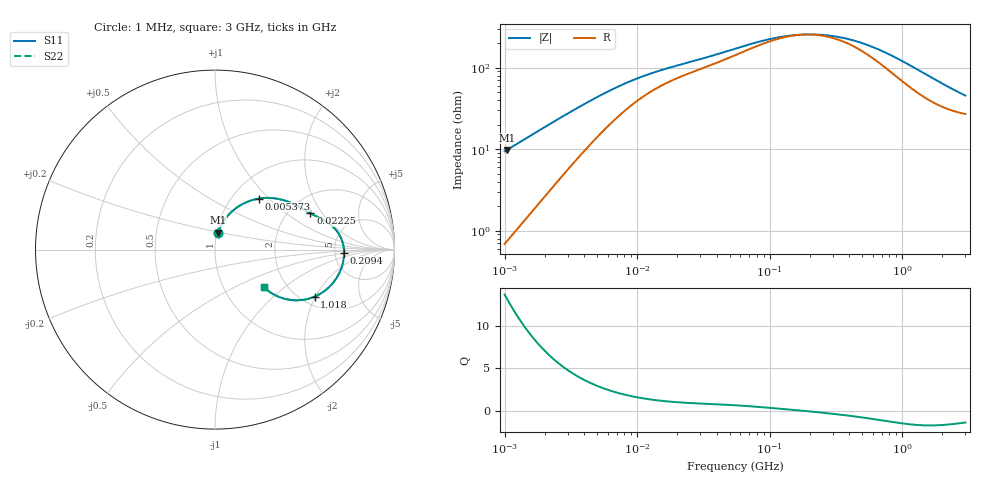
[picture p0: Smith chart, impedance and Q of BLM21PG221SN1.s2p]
! BLM21PG221SN1
# Hz S RI R 50
!Freq.(Hz) S11(Real) S11(Imag) S21(Real) S21(Imag) S12(Real) S12(Imag) S22(Real) S22(Imag)
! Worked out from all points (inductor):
!   401 points, 1 MHz to 3 GHz, reference 50 ohm
!   read as one part in series: L = 1.48 uH near 1.041 MHz
!   highest Q = 13.1 at 1.041 MHz (marker M1), where L = 1.49 uH
!   self-resonance near 183.2 MHz
!   S11 on the Smith chart (normalised r, x): 1 MHz: 1.01, +0.19; 5.373 MHz: 1.32, +0.87; 22.25 MHz: 2.60, +1.56; 209.4 MHz: 6.09, -0.44; 1.018 GHz: 2.34, -1.96; 3 GHz: 1.54, -0.73
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1000000  0.0153 0.0916  0.9847 -0.0916  0.9847 -0.0916  0.0153 0.0916
1040844  0.0166 0.0951  0.9834 -0.0951  0.9834 -0.0951  0.0166 0.0951
2139570  0.0629 0.1787  0.9371 -0.1787  0.9371 -0.1787  0.0629 0.1787
2888807  0.1043 0.221  0.8957 -0.221  0.8957 -0.221  0.1043 0.221
3823119  0.1593 0.2569  0.8407 -0.2569  0.8407 -0.2569  0.1593 0.2569
5372736  0.2441 0.2843  0.7559 -0.2843  0.7559 -0.2843  0.2441 0.2843
8513927  0.3649 0.2797  0.6351 -0.2797  0.6351 -0.2797  0.3649 0.2797
1.461624e7  0.473 0.236  0.527 -0.236  0.527 -0.236  0.473 0.236
2.225279e7  0.5314 0.2027  0.4686 -0.2027  0.4686 -0.2027  0.5314 0.2027
5.477226e7  0.6418 0.1402  0.3582 -0.1402  0.3582 -0.1402  0.6418 0.1402
1.171891e8  0.7054 0.0562  0.2946 -0.0562  0.2946 -0.0562  0.7054 0.0562
1.582265e8  0.7159 0.0187  0.2841 -0.0187  0.2841 -0.0187  0.7159 0.0187
2.094008e8  0.7191 -0.0174  0.2809 0.0174  0.2809 0.0174  0.7191 -0.0174
2.884452e8  0.7152 -0.0614  0.2848 0.0614  0.2848 0.0614  0.7152 -0.0614
3.894533e8  0.7028 -0.1067  0.2972 0.1067  0.2972 0.1067  0.7028 -0.1067
5.696638e8  0.6688 -0.1706  0.3312 0.1706  0.3312 0.1706  0.6688 -0.1706
8.005644e8  0.6125 -0.2287  0.3875 0.2287  0.3875 0.2287  0.6125 -0.2287
1.017911e9  0.555 -0.2621  0.445 0.2621  0.445 0.2621  0.555 -0.2621
1.294266e9  0.4855 -0.2806  0.5145 0.2806  0.5145 0.2806  0.4855 -0.2806
1.645649e9  0.4125 -0.2792  0.5875 0.2792  0.5875 0.2792  0.4125 -0.2792
2.266846e9  0.3272 -0.2496  0.6728 0.2496  0.6728 0.2496  0.3272 -0.2496
3e9  0.2729 -0.2097  0.7271 0.2097  0.7271 0.2097  0.2729 -0.2097
